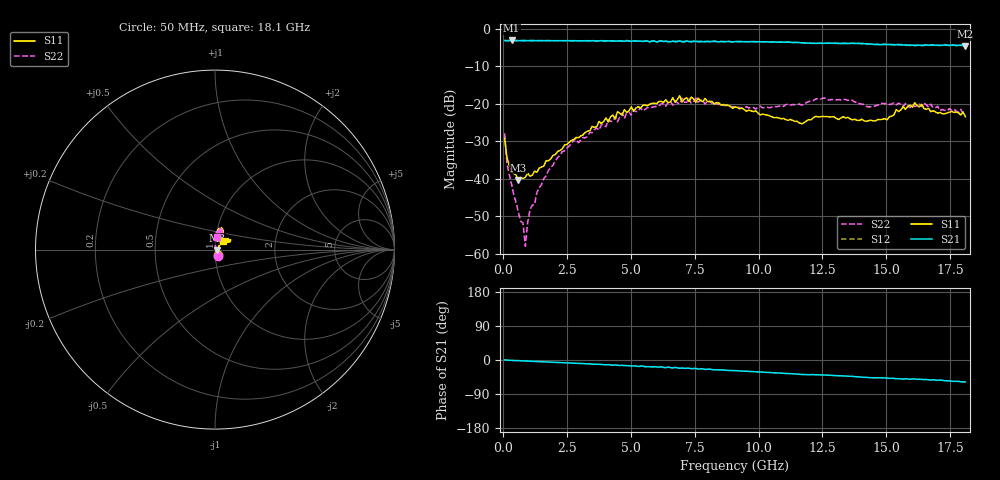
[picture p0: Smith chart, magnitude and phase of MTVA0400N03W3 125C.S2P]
! Network Analyzer HP8720D.06.14 Serial No. US36140669
!  7 Jul 2005  13:51:33
! Frequency  S11  S21  S12  S22
# HZ  S  DB R 50
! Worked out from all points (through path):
!   201 points, 50 MHz to 18.1 GHz, reference 50 ohm
!   highest |S21| = -3.06 dB at 320.8 MHz (marker M1); lowest = -4.6 dB at 18.1 GHz (marker M2)
!   group delay of S21, straight-line fit = 8.88 ps
!   lowest |S11| = -40.3 dB at 591.5 MHz (marker M3), VSWR 1.02, Z = 50.9 - j0.303 ohm
!   |S11| at or under -10 dB: start of sweep to end of sweep
!   |S22| runs from -58.0 to -18.4 dB; largest |S21 - S12| = 0.025
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5e7  -29.13 -64.7  -3.07 0.3  -3.09 0.4  -27.85 -61.2
1.4025e8  -34.28 -53.7  -3.13 -0.3  -3.11 -0.3  -35.81 -69.9
3.2075e8  -38.26 -35.7  -3.06 -0.8  -3.08 -0.8  -41.40 -59.1
5.915e8  -40.34 -18.0  -3.09 -1.6  -3.11 -1.7  -48.96 -31.2
7.72e8  -39.93 -3.0  -3.10 -2.5  -3.09 -2.4  -51.80 -5.6
8.6225e8  -39.60 -3.0  -3.10 -2.5  -3.12 -2.6  -57.98 58.4
1.04275e9  -39.31 10.2  -3.10 -3.3  -3.10 -3.2  -48.23 48.7
1.58425e9  -36.63 19.3  -3.12 -4.9  -3.12 -4.9  -39.94 78.5
2.30625e9  -32.00 35.0  -3.14 -7.1  -3.13 -7.2  -32.75 82.6
3.1185e9  -28.30 50.8  -3.14 -9.3  -3.17 -9.6  -28.98 88.5
4.11125e9  -24.84 58.5  -3.15 -12.1  -3.19 -13.0  -24.17 83.2
4.47225e9  -22.07 57.1  -3.24 -13.8  -3.15 -13.3  -24.78 87.5
4.65275e9  -23.02 58.3  -3.27 -13.9  -3.16 -14.7  -22.44 86.9
6.09675e9  -19.35 67.4  -3.27 -18.8  -3.19 -18.8  -20.56 77.2
6.909e9  -17.82 73.7  -3.14 -22.0  -3.23 -20.9  -19.99 72.4
7.54075e9  -19.56 72.8  -3.32 -22.1  -3.19 -24.1  -18.42 76.7
9.075e9  -20.81 84.0  -3.36 -28.1  -3.34 -28.2  -20.76 67.9
1.169225e10  -25.32 71.2  -3.68 -38.2  -3.68 -38.1  -20.34 71.6
1.21435e10  -23.66 69.9  -3.83 -38.5  -3.79 -38.8  -19.12 74.7
1.512175e10  -23.41 41.0  -4.15 -48.5  -4.03 -48.2  -20.14 80.4
1.61145e10  -19.70 31.4  -4.46 -50.1  -4.22 -50.5  -20.72 76.5
1.81e10  -23.42 47.7  -4.57 -57.7  -4.64 -58.6  -22.95 80.3
